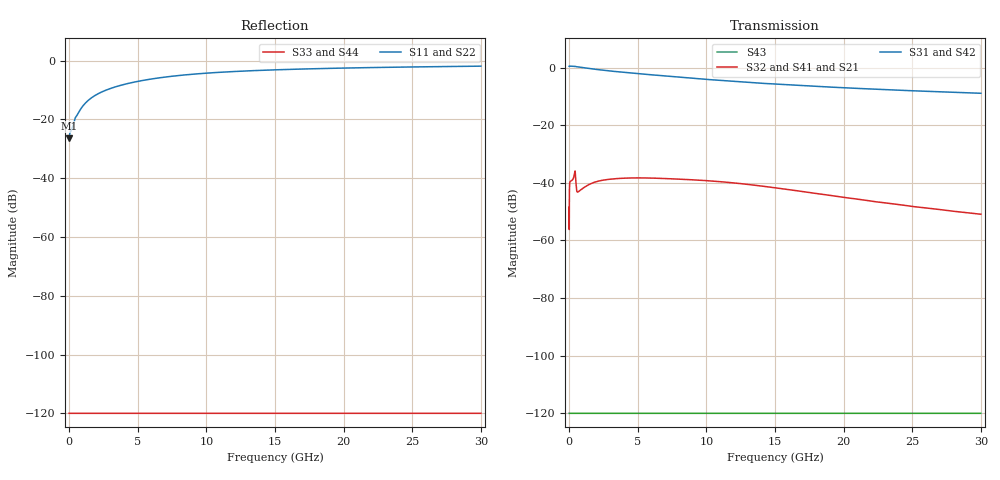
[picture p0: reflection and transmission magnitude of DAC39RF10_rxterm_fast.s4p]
! Copyright 2008, Texas Instruments Incorporated. All rights reserved.
! Generated by program util_convert_RxTerm_to_s4p on 03-29-2011 13:59:36
!  1 ----xxxxxxxxxxxxxxxxxx---- 3
!  xxxxxxxxxxxxxxxxxx
!  (Input) xxxxxxxxxxxxxxxxxx  (Output)
!  xxxxxxxxxxxxxxxxxx
!  2 ----xxxxxxxxxxxxxxxxxx---- 4
! FREQ  S11  S12  S13  S14
!  S21  S22  S23  S24
!  S31  S32  S33  S34
!  S41  S42  S43  S44
!  DB  ANG  DB  ANG  DB  ANG  DB  ANG
# HZ S DB R 50.00
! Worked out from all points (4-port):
!   3000 points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, 10 MHz to 30 GHz, reference 50 ohm
!   strongest paths, dB at 10 MHz, 7.51 GHz, 15.01 GHz, 22.51 GHz, 30 GHz:
!     S31: 0.4, -3.1, -5.7, -7.6, -8.9
!     S42: 0.4, -3.1, -5.8, -7.6, -8.9
!     S32: -48.4, -38.6, -41.7, -46.7, -50.9
!     S41: -48.4, -38.8, -41.8, -46.7, -50.9
!     S21: -48.4, -38.8, -41.8, -46.7, -50.9
!     S43: -120.0, -120.0, -120.0, -120.0, -120.0
!   lowest |S11| = -26.4 dB at 20 MHz (marker M1), VSWR 1.10, Z = 55 - j0.34 ohm
!   |S11| at or under -10 dB: start of sweep to 2.734 GHz
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1e7  -25.62 -4.3  -48.44 -27.9  -120.00 0.0  -120.00 0.0
     -48.38 -28.3  -25.60 -4.3  -120.00 0.0  -120.00 0.0
     0.44 -0.2  -48.44 -27.9  -120.00 0.0  -120.00 0.0
     -48.38 -28.3  0.44 -0.2  -120.00 0.0  -120.00 0.0
2e7  -26.39 -3.7  -56.22 126.0  -120.00 0.0  -120.00 0.0
     -56.58 129.4  -26.35 -3.6  -120.00 0.0  -120.00 0.0
     0.41 -0.2  -56.22 126.0  -120.00 0.0  -120.00 0.0
     -56.58 129.4  0.41 -0.2  -120.00 0.0  -120.00 0.0
3.3e8  -21.60 -52.4  -38.25 4.5  -120.00 0.0  -120.00 0.0
       -38.29 5.0  -21.52 -52.4  -120.00 0.0  -120.00 0.0
       0.45 -3.6  -38.25 4.5  -120.00 0.0  -120.00 0.0
       -38.29 5.0  0.45 -3.6  -120.00 0.0  -120.00 0.0
7e8  -17.65 -83.0  -43.02 -6.8  -120.00 0.0  -120.00 0.0
     -43.01 -7.4  -17.52 -83.1  -120.00 0.0  -120.00 0.0
     0.21 -7.3  -43.02 -6.8  -120.00 0.0  -120.00 0.0
     -43.01 -7.4  0.21 -7.4  -120.00 0.0  -120.00 0.0
1.65e9  -12.64 -108.4  -40.16 5.3  -120.00 0.0  -120.00 0.0
        -40.21 5.0  -12.54 -109.1  -120.00 0.0  -120.00 0.0
        -0.42 -13.4  -40.16 5.3  -120.00 0.0  -120.00 0.0
        -40.21 5.0  -0.45 -13.6  -120.00 0.0  -120.00 0.0
5.69e9  -6.51 -133.0  -38.32 -28.1  -120.00 0.0  -120.00 0.0
        -38.44 -28.4  -6.50 -133.2  -120.00 0.0  -120.00 0.0
        -2.38 -27.0  -38.32 -28.1  -120.00 0.0  -120.00 0.0
        -38.44 -28.4  -2.40 -27.0  -120.00 0.0  -120.00 0.0
3e10  -1.92 -160.8  -50.92 -131.7  -120.00 0.0  -120.00 0.0
      -50.89 -130.9  -1.93 -160.9  -120.00 0.0  -120.00 0.0
      -8.92 -47.4  -50.92 -131.7  -120.00 0.0  -120.00 0.0
      -50.89 -130.9  -8.94 -47.1  -120.00 0.0  -120.00 0.0
